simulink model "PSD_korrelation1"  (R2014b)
settings: Solver=ode45  StartTime=0.0  StopTime=10  RelTol=1e-3
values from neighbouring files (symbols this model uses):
  h = 1    [fourier_reihe_DFT_1.m]    (also in fourier_reihe_rechteck_1.m; fourier_reihe_rechteck_2.m; fourier_transf_puls_1.m; fourier_transf_puls_2.m = 2)
  lag_max = 64    [PSD_korrelation_1.m]
  Ts = 1/fs    (= 0.00025)    [abtast_rate_1.m]    (also in ad_test_12.m = 0.0009765625; ad_test_2.m = 0.00048828125; ad_test_3.m = 0.00048828125; DA_wandler_spektr_1.m = 0.01)
undefined symbols (not defined in the file or in its folder): Fs, get
libraries: dspstat3 x2, dspxfrm3 x1, dspsnks4 x1

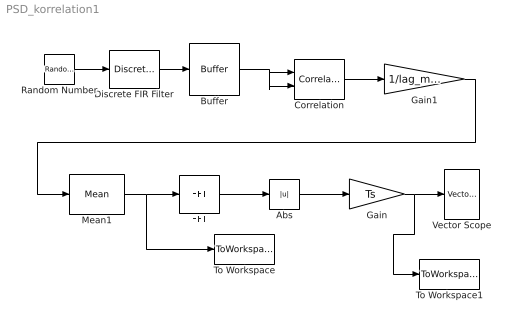
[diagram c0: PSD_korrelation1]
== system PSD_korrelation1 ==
  Abs : Abs
  Buffer : Buffer  N=lag_max  TreatMby1Signals=One channel
  Correlation : dspstat3/Correlation  domain=Time  outputDataTypeStr=Inherit: Same as accumulator  outputLastDataTypeStr=Inherit: Same as accumulator  outputMin=[]  outputMax=[]  roundingMode=Floor  overflowMode=off
  Discrete FIR Filter : DiscreteFir  Coefficients=h
  FFT : dspxfrm3/FFT  CompMethod=Table lookup  TableOpt=NEW  TableOptActive=Speed  BitRevOrder=off  InheritFFTLength=off  FFTLength=nfft  WrapInput=on  RowConvenienceOn=on  FFTImplementation=Auto  SkipNorm=off  firstCoeffDataTypeStr=Inherit: Same word length as input  firstCoeffLastDataTypeStr=Inherit: Same word length as input  outputMin=[]  outputMax=[]  roundingMode=Floor  overflowMode=off
  Gain : Gain  Gain=Ts
  Gain1 : Gain  Gain=1/lag_max
  Mean1 : dspstat3/Mean  run=on  reset_popup=None  directionMode=Each column  dimension=1  treatSBRowAsCol=on  roiEnable=off  roiType=Rectangles  roiPortion=Entire ROI  roiOutput=Individual statistics for each ROI  roiFlag=off  outputDataTypeStr=Inherit: Same as accumulator  outputLastDataTypeStr=Inherit: Same as accumulator  outputMin=[]  outputMax=[]  roundingMode=Floor  overflowMode=off
  Random Number : RandomNumber  SampleTime=Ts
  To Workspace : ToWorkspace  VariableName=Rxx_sim  SaveFormat=Structure  SampleTime=-1
  To Workspace1 : ToWorkspace  VariableName=Sxx  SaveFormat=Structure  SampleTime=-1
  Vector Scope : dspsnks4/Vector Scope  ScopeProperties=on  Domain=Frequency  HorizSpan=1  DisplayProperties=off  AxisGrid=on  Memory=off  FrameNumber=on  AxisLegend=off  AxisZoom=off  OpenScopeAtSimStart=on  OpenScopeImmediately=off  FigPos=get(0,'defaultfigureposition')  AxisProperties=off  XUnits=Hertz  XRange=[-Fs/2...Fs/2]  InheritXIncr=off  XIncr=Ts  XLabel=Time  XLimit=User-defined  XMin=-500  XMax=500  XStart=0  YUnits=dB  YLabel=dBW  LineProperties=off  XAxisParamsVer=6.9
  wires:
  Random Number/1 -> Discrete FIR Filter/1
  Discrete FIR Filter/1 -> Buffer/1
  Buffer/1 -> Correlation/2, Correlation/1
  FFT/1 -> Abs/1
  Abs/1 -> Gain/1
  Gain/1 -> To Workspace1/1, Vector Scope/1
  Correlation/1 -> Gain1/1
  Mean1/1 -> To Workspace/1, FFT/1
  Gain1/1 -> Mean1/1
